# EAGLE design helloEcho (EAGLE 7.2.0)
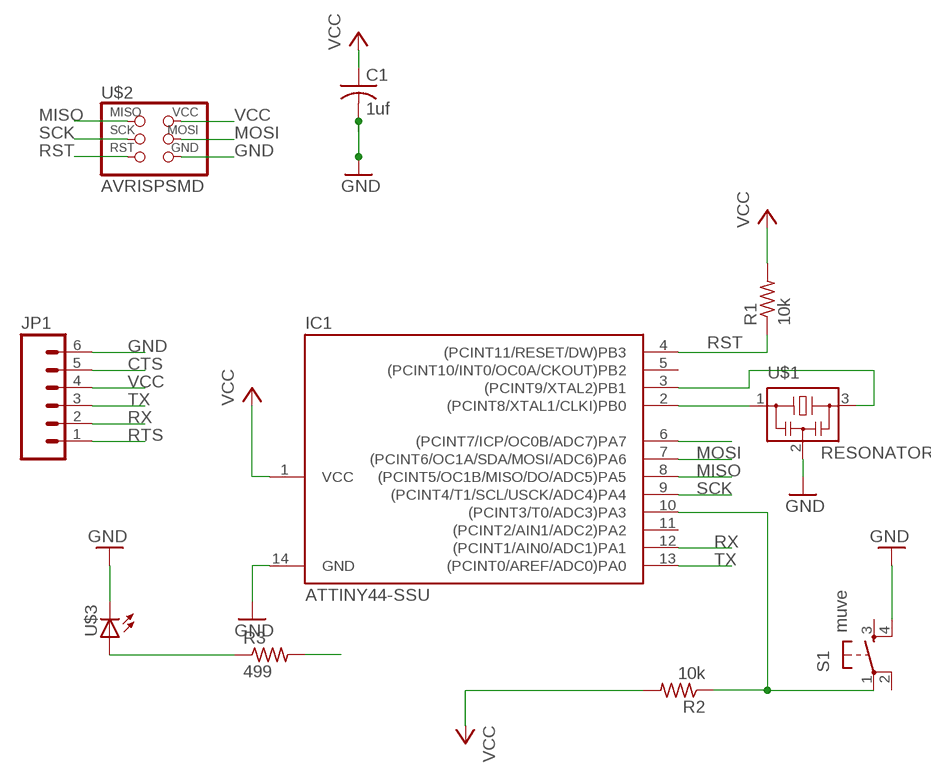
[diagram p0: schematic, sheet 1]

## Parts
C1  1uf  C-USC1206  [C1206]
IC1  ATTINY44-SSU  [SOIC14]
JP1  M06SMD  [1X06-SMD]
R1  10k  R-US_R1206  [R1206]
R2  10k  RESISTOR1206  [1206]
R3  499  RESISTOR1206  [1206]
S1  muve  6MM_SWITCH6MM_SWITCH  [6MM_SWITCH]
U$1  RESONATOR  [EFOBM]
U$2  AVRISPSMD  [2X03SMD]
U$3  LED1206  [1206]

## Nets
CTS: JP1.5
GND: C1.2 IC1.14(GND) JP1.6 S1.4(S1) U$1.2 U$2.6(GND)
LED: IC1.6((PCINT7/ICP/OC0B/ADC7)PA7) R3.2
MISO: IC1.8((PCINT5/OC1B/MISO/DO/ADC5)PA5) U$2.1(MISO)
MOSI: IC1.7((PCINT6/OC1A/SDA/MOSI/ADC6)PA6) U$2.4(MOSI)
N$1: IC1.2((PCINT8/XTAL1/CLKI)PB0) U$1.1
N$2: IC1.3((PCINT9/XTAL2)PB1) U$1.3
N$3: IC1.10((PCINT3/T0/ADC3)PA3) R2.1 S1.1(P)
N$4: U$3.2(C) ; supply symbol labelled GND
N$5: R3.1 U$3.1(A)
RST: IC1.4((PCINT11/RESET/DW)PB3) R1.1 U$2.5(RST)
RTS: JP1.1
RX: IC1.12((PCINT1/AIN0/ADC1)PA1) JP1.2
SCK: IC1.9((PCINT4/T1/SCL/USCK/ADC4)PA4) U$2.3(SCK)
TX: IC1.13((PCINT0/AREF/ADC0)PA0) JP1.3
VCC: C1.1 IC1.1(VCC) JP1.4 R1.2 R2.2 U$2.2(VCC)
Unconnected: IC1.5((PCINT10/INT0/OC0A/CKOUT)PB2) IC1.11((PCINT2/AIN1/ADC2)PA2) S1.2(P1) S1.3(S)

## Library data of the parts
C1 = rcl:C-US: CAPACITOR, American symbol
IC1 = fab:ATTINY44
JP1 = SparkFun:M06: Header 6 Standard 6-pin 0.1" header. Use with straight break away headers (SKU : PRT-00116), right angle break away headers (PRT-00553), swiss pins (PRT-00743), machine pins (PRT-00117), and female headers (PRT-00115). Molex polarized connector foot print use with SKU : PRT-08094 with associated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
R1 = resistor:R-US_: RESISTOR, American symbol
R2 R3 = 01_ng:RESISTOR
S1 = 01_FAB_Hello:6MM_SWITCH: OMRON SWITCH
U$1 = fab:RESONATOR
U$2 = fab:AVRISP
U$3 = 01_FAB_Hello:LED

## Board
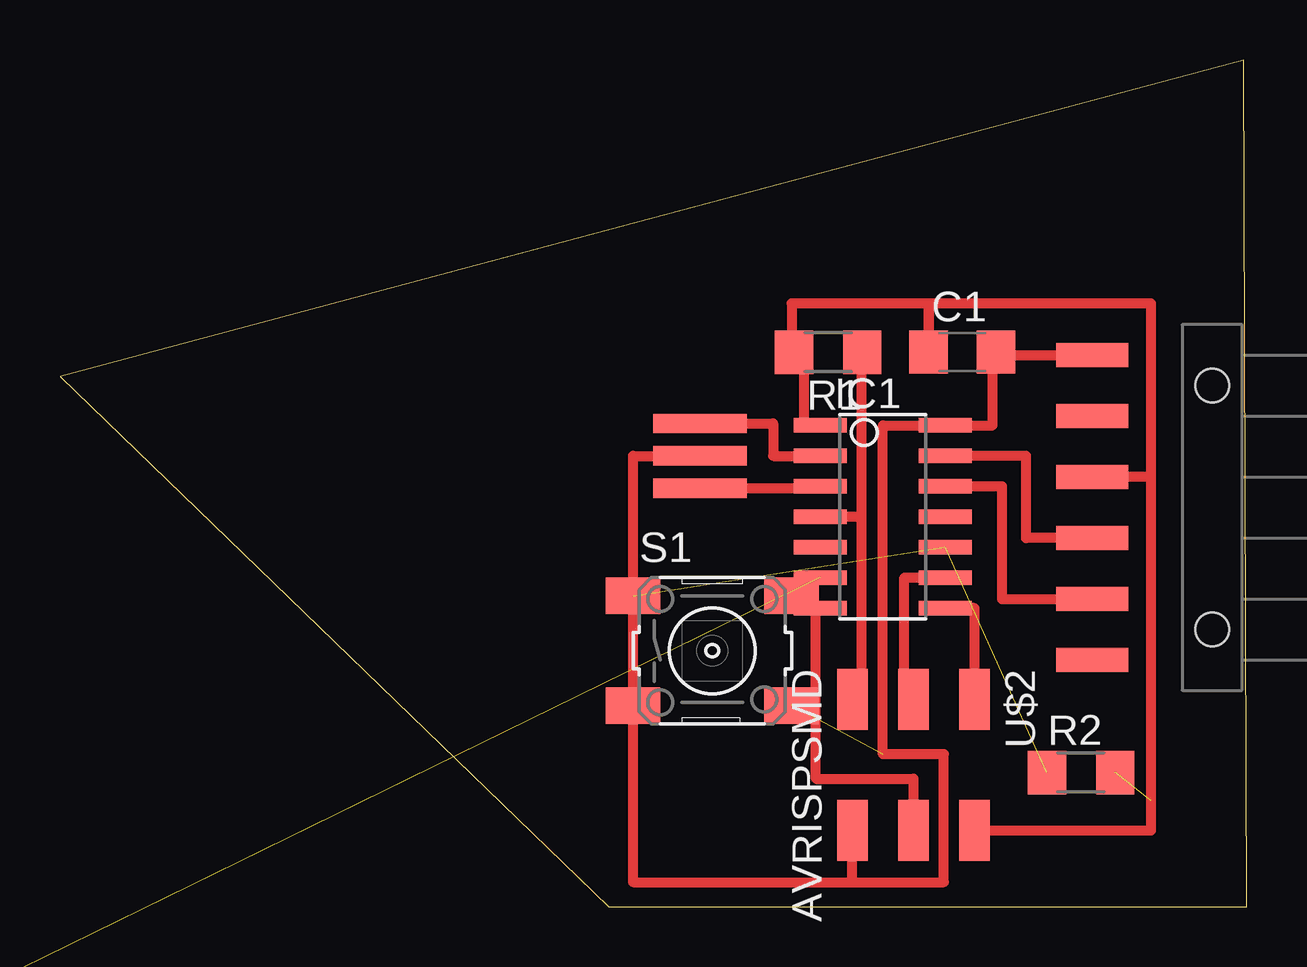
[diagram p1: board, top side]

Size 49.45 x 35.3 mm. Coordinates in mm from the lower left corner, seen from the top.
Outline: 22.86,0 49.45,0 49.33,35.3 0,22.09 22.86,0
Copper layers 1: Top 0.035mm
Design rules "ERP-1sided-10mil-16mill": minimum track width 10mil, minimum drill 24mil, track to track 16mil, track to pad 16mil, pad to pad 16mil, via to via 16mil, smd to smd 0mil, copper to edge 16mil, drill to drill 36mil, minimum pad ring 10mil, minimum via ring 8mil, stop-mask expansion 4mil, vias tented up to drill 0mil, thermal gap 10mil

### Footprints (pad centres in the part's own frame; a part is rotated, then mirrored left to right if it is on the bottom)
C1206 = smd 1.6 x 1.8: 1 -1.4,0; 2 1.4,0
SOIC14 = smd 0.61 x 2.21: 1 -3.81,-2.603; 2 -2.54,-2.603; 3 -1.27,-2.603; 4 0,-2.603; 5 1.27,-2.603; 6 2.54,-2.603; 7 3.81,-2.603; 8 3.81,2.603; 9 2.54,2.603; 10 1.27,2.603; 11 0,2.603; 12 -1.27,2.603; 13 -2.54,2.603; 14 -3.81,2.603
1X06-SMD = smd 1 x 3: 1 -6.35,5; 2 -3.81,5; 3 -1.27,5; 4 1.27,5; 5 3.81,5; 6 6.35,5 | hole 1.4: -5.08,0; 5.08,0
R1206 = smd 1.6 x 1.803: 1 -1.422,0; 2 1.422,0
1206 = smd 1.6 x 1.803: 1 -1.422,0; 2 1.422,0
6MM_SWITCH = smd 2.286 x 1.524: 1 -3.302,2.286; 2 3.302,2.286; 3 -3.302,-2.286; 4 3.302,-2.286
EFOBM = smd 0.8 x 3.9: 1 -1.35,0; 2 0,0; 3 1.35,0
2X03SMD = smd 2.54 x 1.27: 1 -2.54,2.54; 2 2.92,2.54; 3 -2.54,0; 4 2.92,0; 5 -2.54,-2.54; 6 2.92,-2.54

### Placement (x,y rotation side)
C1  37.59,23.11 0 top
IC1  34.29,16.26 270 top
JP1  48.01,16.64 90 top
R1  32,23.11 180 top
R2  42.55,5.59 0 top
R3  not placed on the board
S1  27.18,10.67 0 top
U$1  26.67,18.8 270 top
U$2  35.56,6.1 270 top
U$3  not placed on the board

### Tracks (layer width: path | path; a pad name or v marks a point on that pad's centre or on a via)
GND  (1 unrouted)
  Top 0.406: 33.02,1.02 36.83,1.02 36.83,6.35 34.29,6.35 34.29,20.07 IC1.14 38.86,20.07 38.86,23.11 C1.2 38.99,22.99 JP1.6 43.01,23.24 | U$1.2 23.88,18.8 23.88,1.02 33.02,1.02 | U$2.6 33.02,1.02
LED  (1 unrouted)
MISO
  Top 0.406: IC1.8 38.1,12.45 U$2.1
MOSI
  Top 0.406: IC1.7 31.5,12.45 31.5,5.33 35.56,5.33 U$2.4
N$1
  Top 0.406: U$1.1 29.72,20.15 29.72,18.8 IC1.2
N$2
  Top 0.406: U$1.3 31.69,17.45 IC1.3
N$3  (2 unrouted)
N$5  (1 unrouted)
RST
  Top 0.406: R1.1 33.4,23.11 33.4,16.26 | IC1.4 33.4,16.26 | U$2.5 33.4,8.64 33.4,16.26
RX
  Top 0.406: IC1.12 39.24,17.53 39.24,12.83 JP1.2
SCK
  Top 0.406: U$2.3 35.18,8.64 35.18,13.72 IC1.9
TX
  Top 0.406: JP1.3 40.26,15.37 40.26,18.8 IC1.13
VCC  (1 unrouted)
  Top 0.254: 45.47,4.32 45.47,4.42
  Top 0.406: 45.47,17.91 JP1.4 | 45.47,17.91 45.47,4.32 45.47,3.18 U$2.2 | IC1.1 30.99,20.07 30.99,23.11 R1.2 30.48,23.11 30.48,25.15 36.19,25.15 C1.1 36.2,25.15 45.47,25.15 45.47,17.91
